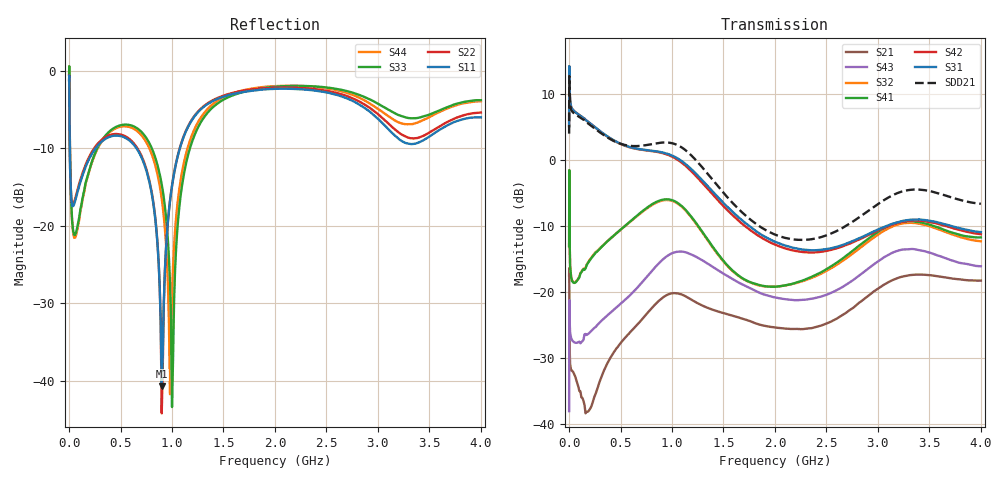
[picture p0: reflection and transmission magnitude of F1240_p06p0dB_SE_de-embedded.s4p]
! Integrated Device Technology
! Corporate Headquarters
! 6024 Silver Creek Valley Road
! San Jose, CA 95138  USA
! Phone:  1-408-284-8200
! Toll Free:  1-800-223-1366
! Webpage:  http://www.idt.com/
! Timing and RF Division
! 515 Groton Road, Suite 102
! Westford, MA 01886-6024
! Device:  F1240
! Description: Dual Intermediate Frequency Digital Variable Gain Amplifier
! Frequency:  10.0 -  500.00 MHz
! Package:  5x5 mm QFN Plastic Package: 32 pin
! Ports:  8 RF, 20 DC
!  Pin  1  = GA3 / Data  Pin 17  = RF OUT_B+
!  Pin  2  = GA4 / CLK  Pin 18  = RF OUT_B-
!  Pin  3  = GA5  Pin 19  = STBY_B
!  Pin  4  = VMODE  Pin 20  = Ground
!  Pin  5  = No Connect  Pin 21  = Ground
!  Pin  6  = GB5  Pin 22  = STB_A
!  Pin  7  = GB4  Pin 23  = RF OUT_A-  = Port 4
!  Pin  8  = GB3  Pin 24  = RF OUT_A+  = Port 3
!  Pin  9  = GB2  Pin 25  = GA0
!  Pin 10  = GB1  Pin 26  = ISET_A
!  Pin 11  = RF IN_B+  Pin 27  = VCC
!  Pin 12  = RF IN_B-  Pin 28  = Ground
!  Pin 13  = Ground  Pin 29  = RF IN_A-  = Port 2
!  Pin 14  = VCC  Pin 30  = RF IN_A+  = Port 1
!  Pin 15  = ISET_B  Pin 31  = GA1
!  Pin 16  = GB0  Pin 32  = GA2 / CSb
! Gain  = +19.5 dB
! State  = 1
! Voltage  = +5.00 V
! Current  = 85.292 mA (one channel only)
! Temperture  =  +25 C
! Test Date  =  2017-10-18
! Board  =  EB4031
! Data:  The device was measured on a custom evaluation board which has
!  individual transmission lines to the RF pins.  Data was collected
!  using a calibrated network analyzer.  The evaluation board was
!  de-embedded using Automatic Fixture Removal.
!  The reference plane is the edge of the package pin.
!  Only Channel A was measured.
!  This data is in single-ended operation.  If your needs are balanced
!  or differential S-parameters then this file needs to be used a
!  linear simulator.
! File Date:  2017-11-10  MJV
! Note:
!  Integrated Device Technology supplies this data as a sample of measured
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# Hz S dB R 100
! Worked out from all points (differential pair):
!   410 points, 500 kHz to 4 GHz, reference 100 ohm
!   strongest paths, dB at 500 kHz, 930 MHz, 1.96 GHz, 2.98 GHz, 4 GHz:
!     S31: 5.1, 1.1, -12.1, -10.7, -10.9
!     S42: 5.1, 0.9, -12.5, -10.8, -11.2
!     S41: -13.0, -6.0, -19.2, -11.1, -11.7
!     S32: -13.1, -6.1, -19.2, -11.5, -12.3
!     S43: -38.0, -14.8, -20.7, -15.6, -16.1
!     S21: -17.5, -20.6, -25.3, -19.7, -18.3
!   taken as a pair (ports 1,2 in; 3,4 out), SDD21 dB: 4.0, 2.7, -11.0, -6.9, -6.6
!   lowest |S11| = -40.8 dB at 900 MHz (marker M1), VSWR 1.02, Z = 98.2 + j0.0873 ohm
!   |S11| at or under -10 dB: 7.538 MHz to 256.6 MHz (249.1 MHz wide, 189 % of centre); 655.1 MHz to 1.076 GHz (421 MHz wide, 48.6 % of centre)
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500000  -1.20 -5.5  -17.47 -5.9  -27.58 82.7  -49.51 77.7
        -17.47 -5.8  -1.20 -5.5  -49.47 76.2  -27.58 83.9
        5.14 -105.2  -13.10 -101.4  -0.48 1.4  -38.06 -76.3
        -13.05 -100.2  5.11 -104.1  -38.02 -76.6  -0.49 3.7
3000000  -3.50 -58.1  -22.40 -71.6  -15.89 26.6  -41.47 -24.3
         -22.44 -71.4  -3.46 -58.1  -41.40 -24.8  -15.90 26.8
         13.28 177.2  -5.26 151.9  -1.88 -57.3  -21.76 -163.2
         -5.33 151.9  13.27 177.4  -21.72 -163.3  -1.93 -57.1
3e7  -17.39 -98.9  -31.92 -18.9  -16.17 -8.0  -48.93 39.2
     -31.92 -19.5  -17.20 -99.4  -48.96 40.2  -16.16 -8.0
     7.71 161.9  -18.27 133.1  -19.38 -117.2  -27.38 161.1
     -18.34 133.6  7.75 161.9  -27.29 161.2  -19.62 -117.7
1.9e8  -11.50 -133.6  -38.06 -7.1  -17.67 -48.7  -35.48 22.9
       -38.01 -5.4  -11.23 -134.6  -35.49 23.7  -17.69 -48.9
       5.73 112.0  -15.35 41.9  -13.06 -114.2  -26.46 102.8
       -15.44 42.1  5.71 111.3  -26.28 102.6  -13.17 -113.2
5.2e8  -8.48 -178.0  -27.68 -22.1  -18.87 -109.5  -29.78 -54.9
       -27.36 -22.2  -8.29 -179.4  -29.91 -52.6  -18.99 -109.8
       2.34 26.7  -10.31 -57.9  -6.96 -163.8  -21.95 11.9
       -10.28 -58.9  2.29 25.8  -21.52 11.7  -7.16 -163.9
9e8  -40.75 177.2  -21.15 -95.1  -17.25 166.4  -27.08 -140.9
     -20.96 -98.8  -44.22 109.3  -27.23 -134.3  -17.54 165.4
     1.17 -69.1  -6.16 -173.5  -14.67 134.4  -15.71 -78.1
     -6.05 -176.7  1.08 -71.0  -15.21 -79.1  -16.50 135.7
4e9  -6.01 -144.2  -18.34 94.7  -21.97 -66.4  -23.00 -46.8
     -18.26 94.1  -5.37 -142.9  -23.82 -28.8  -23.48 -60.3
     -10.92 23.7  -12.31 -89.7  -3.78 -138.6  -17.22 75.6
     -11.73 -103.9  -11.23 30.1  -16.10 58.9  -3.91 -147.0
